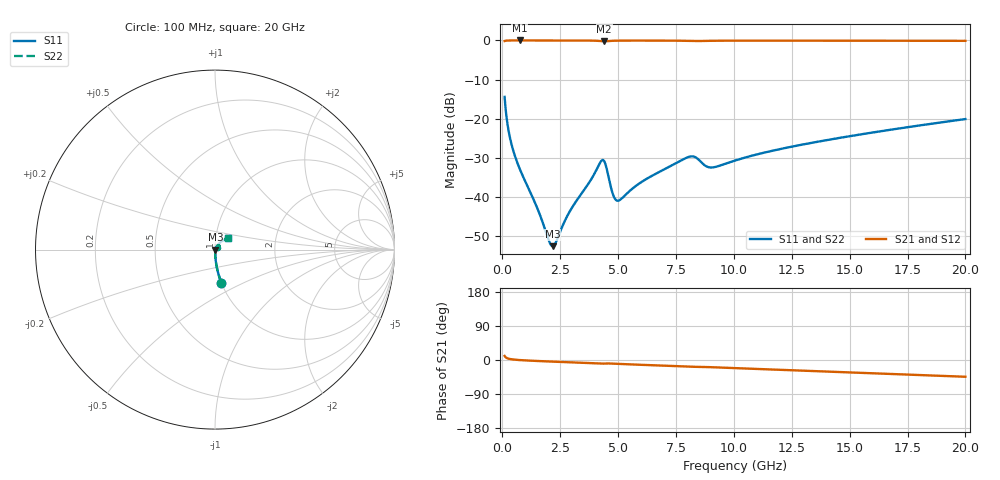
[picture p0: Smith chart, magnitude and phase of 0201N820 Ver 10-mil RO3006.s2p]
# GHz S MA R 50
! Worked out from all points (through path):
!   1601 points, 100 MHz to 20 GHz, reference 50 ohm
!   highest |S21| = -0.01 dB at 746.8 MHz (marker M1); lowest = -0.2 dB at 4.403 GHz (marker M2)
!   group delay of S21, straight-line fit = 6.26 ps
!   lowest |S11| = -52.6 dB at 2.177 GHz (marker M3), VSWR 1.00, Z = 50.2 - j0.0333 ohm
!   |S11| at or under -10 dB: start of sweep to end of sweep
!   |S22| runs from -52.6 to -14.4 dB; largest |S21 - S12| = 0
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0.1  0.1897 -79.0  0.981 10.7  0.981 10.7  0.1897 -79.0
0.2616875  0.07279 -85.6  0.9964 3.7  0.9964 3.7  0.07279 -85.6
0.3611875  0.05216 -86.6  0.9976 2.3  0.9976 2.3  0.05216 -86.6
0.522875  0.03502 -87.2  0.9982 1.0  0.9982 1.0  0.03502 -87.2
0.74675  0.0231 -86.8  0.9984 -0.2  0.9984 -0.2  0.0231 -86.8
1.517875  0.007112 -76.9  0.998 -2.6  0.998 -2.6  0.007112 -76.9
2.027813  0.002693 -37.3  0.9977 -3.9  0.9977 -3.9  0.002693 -37.3
2.177062  0.002351 -8.1  0.9976 -4.3  0.9976 -4.3  0.002351 -8.1
2.326312  0.002683 19.7  0.9975 -4.7  0.9975 -4.7  0.002683 19.7
2.886  0.006322 56.9  0.997 -6.1  0.997 -6.1  0.006322 56.9
3.420812  0.01103 63.3  0.9962 -7.4  0.9962 -7.4  0.01103 63.3
4.241688  0.02796 39.9  0.9815 -9.6  0.9815 -9.6  0.02796 39.9
4.403375  0.02857 13.7  0.9735 -9.4  0.9735 -9.4  0.02857 13.7
4.7765  0.01083 0.6  0.9892 -9.6  0.9892 -9.6  0.01083 0.6
4.9755  0.008955 23.4  0.9924 -10.1  0.9924 -10.1  0.008955 23.4
6.741625  0.0206 61.0  0.9945 -14.5  0.9945 -14.5  0.0206 61.0
8.122188  0.03288 46.5  0.9851 -17.7  0.9851 -17.7  0.03288 46.5
8.980375  0.0238 41.8  0.9879 -18.9  0.9879 -18.9  0.0238 41.8
10.05  0.02918 55.1  0.9926 -21.4  0.9926 -21.4  0.02918 55.1
13.37081  0.04919 53.8  0.9923 -29.0  0.9923 -29.0  0.04919 53.8
16.69162  0.07167 48.0  0.9903 -36.5  0.9903 -36.5  0.07167 48.0
20  0.09887 41.4  0.9871 -44.2  0.9871 -44.2  0.09887 41.4
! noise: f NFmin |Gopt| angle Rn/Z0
0.1  0.0005794  0.9261  0.2313  0.001739
2.301  0.004675  0.8029  4.568  0.004916
4.515  0.01999  0.9047  8.951  0.04571
6.729  0.01165  0.7737  13.27  0.01037
8.943  0.02054  0.8254  17.62  0.02415
11.14  0.01632  0.7404  21.82  0.01215
13.36  0.01792  0.7218  26.01  0.01214
15.57  0.01989  0.7119  30.14  0.01271
17.79  0.02193  0.7053  34.21  0.01338
20  0.02398  0.7008  38.21  0.01406
